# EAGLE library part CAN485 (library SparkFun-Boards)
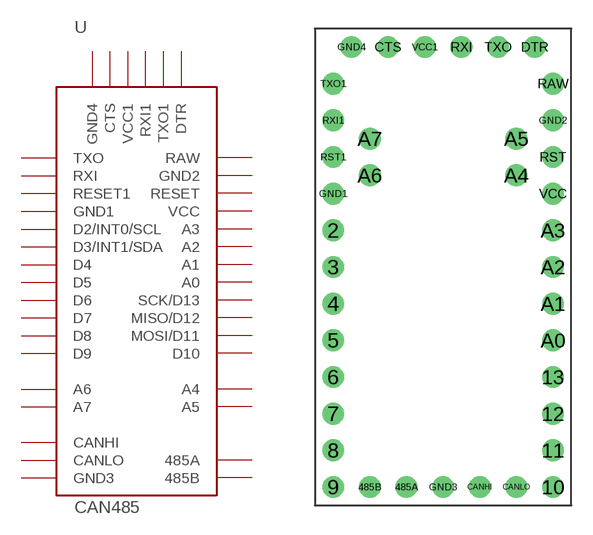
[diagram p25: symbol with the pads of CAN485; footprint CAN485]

Designator prefix -

## CAN485FULL_SOCKET  [CAN485]
2  D2/INT0/SCL
3  D3/INT1/SDA
4  D4
5  D5
6  D6
7  D7
8  D8
9  D9
10  D10
11  MOSI/D11
12  MISO/D12
13  SCK/D13
485A  485A
485B  485B
A0  A0
A1  A1
A2  A2
A3  A3
A4  A4
A5  A5
A6  A6
A7  A7
CANHI  CANHI
CANLO  CANLO
CTS  CTS
DTR  DTR
GND1  GND1
GND2  GND2
GND3  GND3
GND4  GND4
RAW  RAW
RST  RESET
RST1  RESET1
RXI  RXI
RXI1  RXI1
TXO  TXO
TXO1  TXO1
VCC  VCC
VCC1  VCC1

## Footprint CAN485 (pad centres in mm)
drill 1: 2 -7.62,2.54; 3 -7.62,0; 4 -7.62,-2.54; 5 -7.62,-5.08; 6 -7.62,-7.62; 7 -7.62,-10.16; 8 -7.62,-12.7; 9 -7.62,-15.24; 10 7.62,-15.24; 11 7.62,-12.7; 12 7.62,-10.16; 13 7.62,-7.62; 485A -2.54,-15.24; 485B -5.08,-15.24; A0 7.62,-5.08; A1 7.62,-2.54; A2 7.62,0; A3 7.62,2.54; A4 5.08,6.35; A5 5.08,8.89; A6 -5.08,6.35; A7 -5.08,8.89; CANHI 2.54,-15.24; CANLO 5.08,-15.24; CTS -3.81,15.24; DTR 6.35,15.24; GND1 -7.62,5.08; GND2 7.62,10.16; GND3 0,-15.24; GND4 -6.35,15.24; RAW 7.62,12.7; RST 7.62,7.62; RST1 -7.62,7.62; RXI 1.27,15.24; RXI1 -7.62,10.16; TXO 3.81,15.24; TXO1 -7.62,12.7; VCC 7.62,5.08; VCC1 -1.27,15.24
